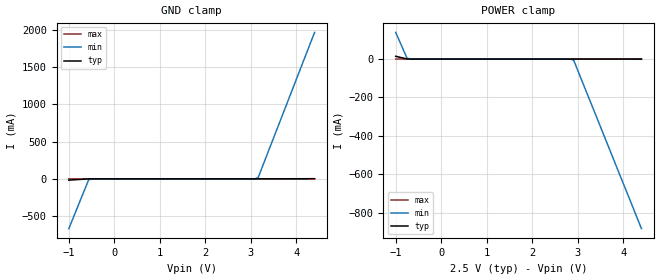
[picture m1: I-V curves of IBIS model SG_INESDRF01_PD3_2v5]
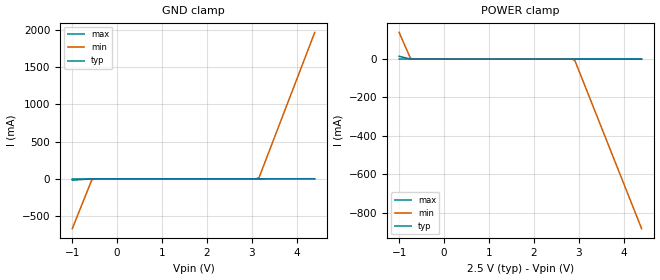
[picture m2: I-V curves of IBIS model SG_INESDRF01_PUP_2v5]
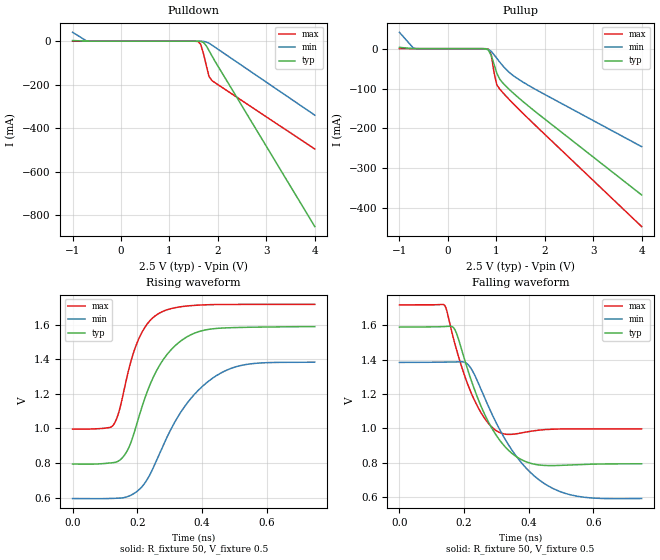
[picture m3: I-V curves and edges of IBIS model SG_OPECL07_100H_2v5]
|   This file is an IBIS representation of the   |
|   Integrated Device Technology , Inc.   |
|   ICS853S01I   |
|   2:1, DIFFERENTIAL TO-LVPECL MULTIPLEXER   |
[IBIS Ver]   4.1
[File name]   853s01i.ibs
[File Rev]   1.0
[Date]   26 May 2010
[Source]   Originated at Integrated Device Technology, Inc.
[Disclaimer]
IDT hereby grants the user of this IBIS model a non-exclusive,
nontransferable license to use this IBIS model under the following terms.
Before using this IBIS model, the user should read this license.
If the user does not accept these terms,  the IBIS model should be
returned to IDT within 30 days.
   The user is granted this license only to use the IBIS model and
is not granted rights to sell, load, rent, lease or license the IBIS
model in whole or in part, or in modified form to anyone other than
user. User may modify the IBIS model to suit its specific
applications but rights to derivative works and such modifications
shall belong to IDT.
   This IBIS model is provided on an "AS IS" basis and IDT makes
absolutely no warranty with respect to the information contained
herein. IDT DISCLAIMS AND CUSTOMER WAIVES ALL WARRANTIES, EXPRESS
OR IMPLIED, INCLUDING WARRANTIES OF MERCHANTABILITY OR FITNESS FOR
A PARTICULAR PURPOSE. The entire risk as to quality and performance
is with the Customer. ACCORDINGLY, IN NO EVENT SHALL THE COMPANY BE
LIABLE FOR ANY DAMAGES, WHETHER IN CONTRACT OR TORT,INCLUDING ANY
LOST PROFITS OR OTHER INCIDENTAL, CONSEQUENTIAL, EXEMPLARY, OR
PUNITIVE DAMAGES ARISING OUT OF THE USE OR APPLICATION OF THE IBIS
model provided in this package. Further, IDT reserves the right to
make changes without notice to any product herein to improve
reliability, function, or design. IDT does not convey any license
under patent rights or any other intellectual property rights,
including those of third parties.
   IDT is not obligated to provide maintenance or support
for the licensed IBIS model.
[Copyright]   Copyright 2010 by Integrated Device Technology, Inc.
[Component]   ICS853S01AKI
[Manufacturer] Integrated Device Technology, Inc.
[Package]
|LD QFN 16
|lead + wire   typ   min   max
R_pkg   72.4655m   58.886m   86.045m
L_pkg   1.47175nH   1.11650nH   1.77850nH
C_pkg   0.07747pF   0.07444pF   0.08050pF
[Pin] signal_name   model_name   R_pin   L_pin   C_pin
1   PCLK0   SG_INESDRF01_PD3   86.045m   1.77850nH   0.08050pF
2   nPCLK0   SG_INESDRF01_PUP   58.886m   1.11650nH   0.07444pF
3   PCLK1   SG_INESDRF01_PD3   58.886m   1.11650nH   0.07444pF
4   nPCLK1   SG_INESDRF01_PUP   86.045m   1.77850nH   0.08050pF
5   VBB   GND   86.045m   1.77850nH   0.08050pF
6   CLK_SEL   SG_INESDRF01_PD3   58.886m   1.11650nH   0.07444pF
7   nc   NC   58.886m   1.11650nH   0.07444pF
8   VCC   POWER   86.045m   1.77850nH   0.08050pF
9   VEE   GND   86.045m   1.77850nH   0.08050pF
10  nQ   SG_OPECL07_100H   58.886m   1.11650nH   0.07444pF
11  Q   SG_OPECL07_100H   58.886m   1.11650nH   0.07444pF
12  VEE   GND   86.045m   1.77850nH   0.08050pF
13  VCC   POWER   86.045m   1.77850nH   0.08050pF
14  VEE   GND   58.886m   1.11650nH   0.07444pF
15  VEE   GND   58.886m   1.11650nH   0.07444pF
16  nc   NC   86.045m   1.77850nH   0.08050pF
[Diff Pin]  inv_pin  vdiff   tdelay_typ tdelay_min  tdelay_max
11   10   0.15   0   0   0
1   2   NA   0   0   0
3   4   NA   0   0   0
[Component]   ICS853S01AGI
[Manufacturer] Integrated Device Technology, Inc.
[Package]
|   TSSOP16   typ   min   max
R_pkg   58.65m   52.5m   64.8m
L_pkg   1.902nH   1.443nH   2.361nH
C_pkg   0.315pF   0.254pF   0.375pF
[Pin] signal_name   model_name   R_pin   L_pin   C_pin
1  PCLK0   SG_INESDRF01_PD3   64.8m   2.361n   0.375p
2  nPCLK0   SG_INESDRF01_PUP   60.7m   2.054n   0.335p
3  PCLK1   SG_INESDRF01_PD3   56.6m   1.749n   0.294p
4  nPCLK1   SG_INESDRF01_PUP   52.5m   1.443n   0.254p
5  VBB   GND   52.5m   1.443n   0.254p
6  CLK_SEL   SG_INESDRF01_PD3   56.6m   1.749n   0.294p
7  nc   NC   60.7m   2.054n   0.335p
8  VCC   POWER   64.8m   2.361n   0.375p
9  VEE   GND   64.8m   2.361n   0.375p
10 nQ   SG_OPECL07_100H   60.7m   2.054n   0.335p
11 Q   SG_OPECL07_100H   56.6m   1.749n   0.294p
12 VEE   GND   52.5m   1.443n   0.254p
13 VCC   POWER   52.5m   1.443n   0.254p
14 VEE   GND   56.6m   1.749n   0.294p
15 VEE   GND   60.7m   2.054n   0.335p
16 nc   NC   64.8m   2.361n   0.375p
[Diff Pin]  inv_pin  vdiff   tdelay_typ tdelay_min  tdelay_max
11   10   0.15   0   0   0
1   2   NA   0   0   0
3   4   NA   0   0   0
[Model Selector] SG_INESDRF01_PD3
SG_INESDRF01_PD3_2v5  Buffer selection for 2v5
SG_INESDRF01_PD3_3v3  Buffer selection for 3v3
[Model Selector] SG_INESDRF01_PUP
SG_INESDRF01_PUP_2v5  Buffer selection for 2v5
SG_INESDRF01_PUP_3v3  Buffer selection for 3v3
[Model Selector] SG_OPECL07_100H
SG_OPECL07_100H_2v5  Buffer selection for 2v5
SG_OPECL07_100H_3v3  Buffer selection for 3v3
| Models and submodels in the file (6): SG_INESDRF01_PD3_2v5 (Input), SG_INESDRF01_PUP_2v5 (Input), SG_OPECL07_100H_2v5 (Output_ECL), SG_INESDRF01_PD3_3v3 (Input), SG_INESDRF01_PUP_3v3 (Input), SG_OPECL07_100H_3v3 (Output_ECL)
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[Model] SG_INESDRF01_PD3_2v5
Model_type   Input
Polarity   Non-Inverting
Vinl = 0.7V
Vinh = 1.7V
|   typ   min   max
C_comp   2pF   1.5pF   2.5pF
|   typ   min   max
[Voltage range]   2.5V   2.375V   2.625V
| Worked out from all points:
|   GND clamp passes 1 mA (typ) near -0.58 V on its own axis
|   POWER clamp passes 1 mA (typ) near -0.76 V on its own axis
[GND_clamp]
|Voltage   I (typ)   I (min)   I (max)
-999mV    -17.26mA   -669.4mA   -69.92uA
-564.6mV  -253uA     -14.48mA   -14.25uA
-502.5mV  -34.49uA   -1.95mA    -12.42uA
3.035V    79.9uA     353.1uA    74.94uA
3.159V    92.75uA    15.18mA    78.01uA
4.4V      2.096mA    1.969A     108.7uA
[Power_clamp]
|Voltage   I (typ)   I (min)   I (max)
-999mV    14.55mA    139mA      455.8uA
-750.8mV  431.5uA    5.254mA    87.68uA
-688.7mV  114.8uA    775.3uA    82.03uA
2.787V    -7.54uA    -112.5uA   -3.988uA
2.911V    -11.39uA   -5.67mA    -7.053uA
4.4V      -196uA     -883.8mA   -43.83uA
[Model] SG_INESDRF01_PUP_2v5
Model_type   Input
Polarity   Non-Inverting
Vinl = 0.7V
Vinh = 1.7V
|   typ   min   max
C_comp   2pF   1.5pF   2.5pF
|   typ   min   max
[Voltage range]   2.5V   2.375V   2.625V
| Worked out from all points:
|   GND clamp passes 1 mA (typ) near -0.58 V on its own axis
|   POWER clamp passes 1 mA (typ) near -0.76 V on its own axis
[GND_clamp]
|Voltage   I (typ)   I (min)   I (max)
-999mV    -17.36mA   -669.5mA   -167.9uA
-564.6mV  -337.9uA   -14.56mA   -99.91uA
-502.5mV  -117.6uA   -2.03mA    -96.32uA
3.035V    98.13uA    373.4uA    91.38uA
3.159V    114.5uA    15.21mA    97.97uA
4.4V      2.153mA    1.969A     163.9uA
[Power_clamp]
|Voltage   I (typ)   I (min)   I (max)
-999mV    14.58mA    139.1mA    488.9uA
-750.8mV  455.9uA    5.277mA    113.8uA
-688.7mV  137.4uA    796.5uA    106.4uA
2.787V    -84.42uA   -190.4uA   -78.21uA
2.911V    -91.83uA   -5.751mA   -84.8uA
4.4V      -319.1uA   -883.9mA   -163.8uA
[Model] SG_OPECL07_100H_2v5
Model_type   Output_ECL
Polarity   Non-Inverting
|   typ   min   max
C_comp   2pF   1.5pF   2.5pF
Vmeas = 1.22V
Rref = 50
Cref = 0
Vref = 0.5V
|   typ   min   max
[Voltage range]   2.5V   2.375V   2.625V
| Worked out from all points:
|   rising waveform, R_fixture 50, V_fixture 0.5: 20-80 % time 106ps typ, 147ps min, 70.2ps max; typ from 0.794 V to 1.59 V
|   falling waveform, R_fixture 50, V_fixture 0.5: 20-80 % time 105ps typ, 149ps min, 77.6ps max; typ from 1.59 V to 0.794 V
[Pulldown]
|Voltage   I (typ)   I (min)   I (max)
-999mV    3.236mA    41.07mA    51.47uA
-711.7mV  75.61uA    1.458mA    617.8nA
-654.2mV  8.078uA    226.5uA    35.41nA
1.587V    -86.48uA   -19.21uA   -1.152mA
1.644V    -752.2uA   -118.1uA   -13.49mA
1.702V    -5.318mA   -685.4uA   -55.72mA
1.759V    -20.29mA   -3.152mA   -109.3mA
1.817V    -42.51mA   -9.053mA   -161.7mA
1.874V    -65.92mA   -17.23mA   -179.8mA
4V        -852mA     -339.8mA   -495.5mA
[Pullup]
|Voltage   I (typ)   I (min)   I (max)
-999mV    3.236mA    41.07mA    51.47uA
-711.7mV  75.61uA    1.458mA    617.8nA
724.8mV   -60.94uA   -68.32uA   -5.553uA
839.7mV   -4.039mA   -2.1mA     -1.493mA
897.2mV   -17.48mA   -7.16mA    -16.22mA
954.6mV   -39.41mA   -15.28mA   -60.59mA
1.012V    -62.14mA   -24.41mA   -91.49mA
1.07V     -76.16mA   -33.41mA   -101.1mA
1.127V    -84.99mA   -41.9mA    -109.3mA
1.357V    -112.3mA   -68.3mA    -138.8mA
1.702V    -147.8mA   -94.78mA   -180.2mA
4V        -367.2mA   -246mA     -446.5mA
[Ramp]
|   typ   min   max
dV/dt_r   0.636/0.167n   0.631/0.224n   0.577/0.112n
dV/dt_f   0.649/0.158n   0.638/0.221n   0.605/0.118n
R_load =   50.0000
[Rising Waveform]
R_fixture = 50
V_fixture = 0.5   | VCC_typ - 2V
V_fixture_max = 0.625   | VCC_max - 2V
V_fixture_min = 0.375   | VCC_min - 2V
C_fixture = 0.0p
| Time   typ   min   max
0s        794.1mV    594.5mV    996.6mV
120.9ps   801.1mV    594.9mV    1.011V
154.7ps   831.9mV    598.4mV    1.182V
177.9ps   906.2mV    611.4mV    1.371V
205ps     1.065V     644.6mV    1.519V
271.8ps   1.373V     866.2mV    1.671V
354.4ps   1.531V     1.146V     1.709V
453.5ps   1.58V      1.315V     1.718V
550.3ps   1.586V     1.374V     1.718V
749.2ps   1.589V     1.384V     1.718V
[Falling Waveform]
R_fixture = 50
V_fixture = 0.5   | VCC_typ - 2V
V_fixture_max = 0.625   | VCC_max - 2V
V_fixture_min = 0.375   | VCC_min - 2V
C_fixture = 0.0p
| Time   typ   min   max
0s        1.589V     1.384V     1.718V
138.1ps   1.593V     1.385V     1.719V
167.4ps   1.586V     1.386V     1.521V
219.2ps   1.295V     1.355V     1.218V
263.5ps   1.082V     1.178V     1.058V
306.3ps   940.9mV    1.007V     978.9mV
385.1ps   810.5mV    782.6mV    976.1mV
474.5ps   783.2mV    650.3mV    995.1mV
574.3ps   790.4mV    598.3mV    996.8mV
749.2ps   793.7mV    591.6mV    996.5mV
